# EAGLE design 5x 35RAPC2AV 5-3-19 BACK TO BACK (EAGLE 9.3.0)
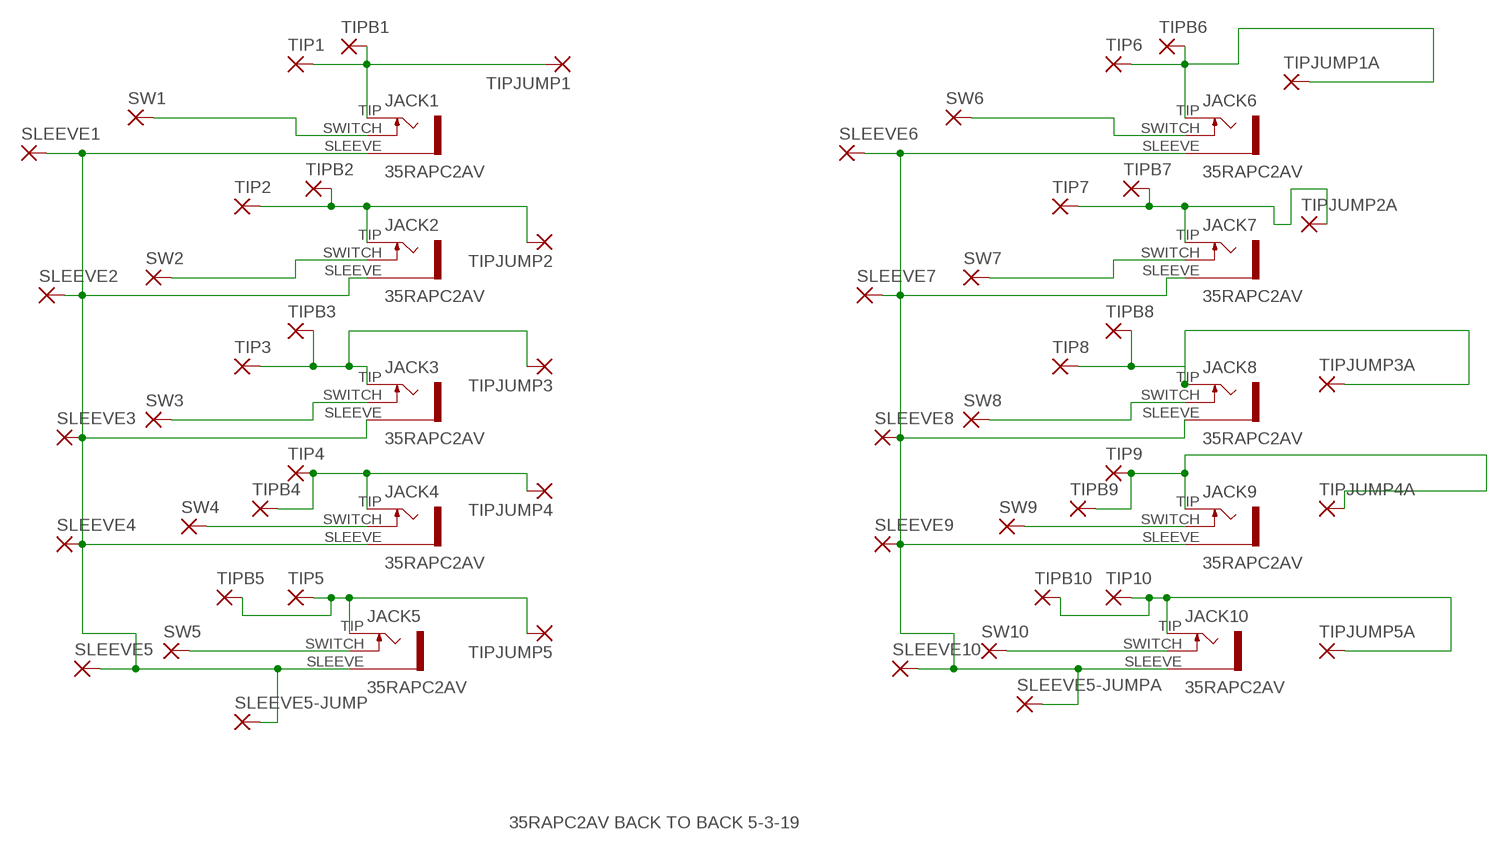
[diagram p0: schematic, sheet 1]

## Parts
JACK1  35RAPC2AV  [35RAPCVAV]
JACK2  35RAPC2AV  [35RAPCVAV]
JACK3  35RAPC2AV  [35RAPCVAV]
JACK4  35RAPC2AV  [35RAPCVAV]
JACK5  35RAPC2AV  [35RAPCVAV]
JACK6  35RAPC2AV  [35RAPCVAV]
JACK7  35RAPC2AV  [35RAPCVAV]
JACK8  35RAPC2AV  [35RAPCVAV]
JACK9  35RAPC2AV  [35RAPCVAV]
JACK10  35RAPC2AV  [35RAPCVAV]
SLEEVE1  2,54/1,1  [2,54/1,1]
SLEEVE2  2,54/1,1  [2,54/1,1]
SLEEVE3  2,54/1,1  [2,54/1,1]
SLEEVE4  2,54/1,1  [2,54/1,1]
SLEEVE5  2,54/1,1  [2,54/1,1]
SLEEVE5-JUMP  2,54/1,1  [2,54/1,1]
SLEEVE5-JUMPA  2,54/1,1  [2,54/1,1]
SLEEVE6  2,54/1,1  [2,54/1,1]
SLEEVE7  2,54/1,1  [2,54/1,1]
SLEEVE8  2,54/1,1  [2,54/1,1]
SLEEVE9  2,54/1,1  [2,54/1,1]
SLEEVE10  2,54/1,1  [2,54/1,1]
SW1  2,54/1,1  [2,54/1,1]
SW2  2,54/1,1  [2,54/1,1]
SW3  2,54/1,1  [2,54/1,1]
SW4  2,54/1,1  [2,54/1,1]
SW5  2,54/1,1  [2,54/1,1]
SW6  2,54/1,1  [2,54/1,1]
SW7  2,54/1,1  [2,54/1,1]
SW8  2,54/1,1  [2,54/1,1]
SW9  2,54/1,1  [2,54/1,1]
SW10  2,54/1,1  [2,54/1,1]
TIP1  2,54/1,1  [2,54/1,1]
TIP2  2,54/1,1  [2,54/1,1]
TIP3  2,54/1,1  [2,54/1,1]
TIP4  2,54/1,1  [2,54/1,1]
TIP5  2,54/1,1  [2,54/1,1]
TIP6  2,54/1,1  [2,54/1,1]
TIP7  2,54/1,1  [2,54/1,1]
TIP8  2,54/1,1  [2,54/1,1]
TIP9  2,54/1,1  [2,54/1,1]
TIP10  2,54/1,1  [2,54/1,1]
TIPB1  2,54/1,1  [2,54/1,1]
TIPB2  2,54/1,1  [2,54/1,1]
TIPB3  2,54/1,1  [2,54/1,1]
TIPB4  2,54/1,1  [2,54/1,1]
TIPB5  2,54/1,1  [2,54/1,1]
TIPB6  2,54/1,1  [2,54/1,1]
TIPB7  2,54/1,1  [2,54/1,1]
TIPB8  2,54/1,1  [2,54/1,1]
TIPB9  2,54/1,1  [2,54/1,1]
TIPB10  2,54/1,1  [2,54/1,1]
TIPJUMP1  2,54/1,1  [2,54/1,1]
TIPJUMP1A  2,54/1,1  [2,54/1,1]
TIPJUMP2  2,54/1,1  [2,54/1,1]
TIPJUMP2A  2,54/1,1  [2,54/1,1]
TIPJUMP3  2,54/1,1  [2,54/1,1]
TIPJUMP3A  2,54/1,1  [2,54/1,1]
TIPJUMP4  2,54/1,1  [2,54/1,1]
TIPJUMP4A  2,54/1,1  [2,54/1,1]
TIPJUMP5  2,54/1,1  [2,54/1,1]
TIPJUMP5A  2,54/1,1  [2,54/1,1]

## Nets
N$2: JACK1.SWITCH SW1.1(P)
N$3: JACK1.SLEEVE JACK2.SLEEVE JACK3.SLEEVE JACK4.SLEEVE JACK5.SLEEVE SLEEVE1.1(P) SLEEVE2.1(P) SLEEVE3.1(P) SLEEVE4.1(P) SLEEVE5-JUMP.1(P) SLEEVE5.1(P)
N$4: JACK2.TIP TIP2.1(P) TIPB2.1(P) TIPJUMP2.1(P)
N$5: JACK6.TIP TIP6.1(P) TIPB6.1(P) TIPJUMP1A.1(P)
N$6: JACK6.SWITCH SW6.1(P)
N$7: JACK6.SLEEVE JACK7.SLEEVE JACK8.SLEEVE JACK9.SLEEVE JACK10.SLEEVE SLEEVE5-JUMPA.1(P) SLEEVE6.1(P) SLEEVE7.1(P) SLEEVE8.1(P) SLEEVE9.1(P) SLEEVE10.1(P)
N$8: JACK3.SWITCH SW3.1(P)
N$9: JACK3.TIP TIP3.1(P) TIPB3.1(P) TIPJUMP3.1(P)
N$10: JACK4.TIP TIP4.1(P) TIPB4.1(P) TIPJUMP4.1(P)
N$11: JACK4.SWITCH SW4.1(P)
N$12: JACK7.TIP TIP7.1(P) TIPB7.1(P) TIPJUMP2A.1(P)
N$13: JACK5.TIP TIP5.1(P) TIPB5.1(P) TIPJUMP5.1(P)
N$14: JACK5.SWITCH SW5.1(P)
N$15: JACK8.SWITCH SW8.1(P)
N$16: JACK8.TIP TIP8.1(P) TIPB8.1(P) TIPJUMP3A.1(P)
N$17: JACK9.TIP TIP9.1(P) TIPB9.1(P) TIPJUMP4A.1(P)
N$18: JACK9.SWITCH SW9.1(P)
N$19: JACK10.TIP TIP10.1(P) TIPB10.1(P) TIPJUMP5A.1(P)
N$20: JACK10.SWITCH SW10.1(P)
SW1: JACK7.SWITCH SW7.1(P)
SW2: JACK2.SWITCH SW2.1(P)
TIP1: JACK1.TIP TIP1.1(P) TIPB1.1(P) TIPJUMP1.1(P)

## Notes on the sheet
- 35RAPC2AV BACK TO BACK 5-3-19

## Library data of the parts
JACK1-JACK10 = MusicThingModular-CL:35RAPC2AV: Switchcraft 35RAPC2AV jack
SLEEVE1-SLEEVE5 SLEEVE5-JUMP SLEEVE5-JUMPA SLEEVE6-SLEEVE10 SW1-SW10 TIP1-TIP10 TIPB1-TIPB10 TIPJUMP1 TIPJUMP1A TIPJUMP2 TIPJUMP2A TIPJUMP3 TIPJUMP3A TIPJUMP4 TIPJUMP4A TIPJUMP5 TIPJUMP5A = wirepad:2,54/1,1: THROUGH-HOLE PAD

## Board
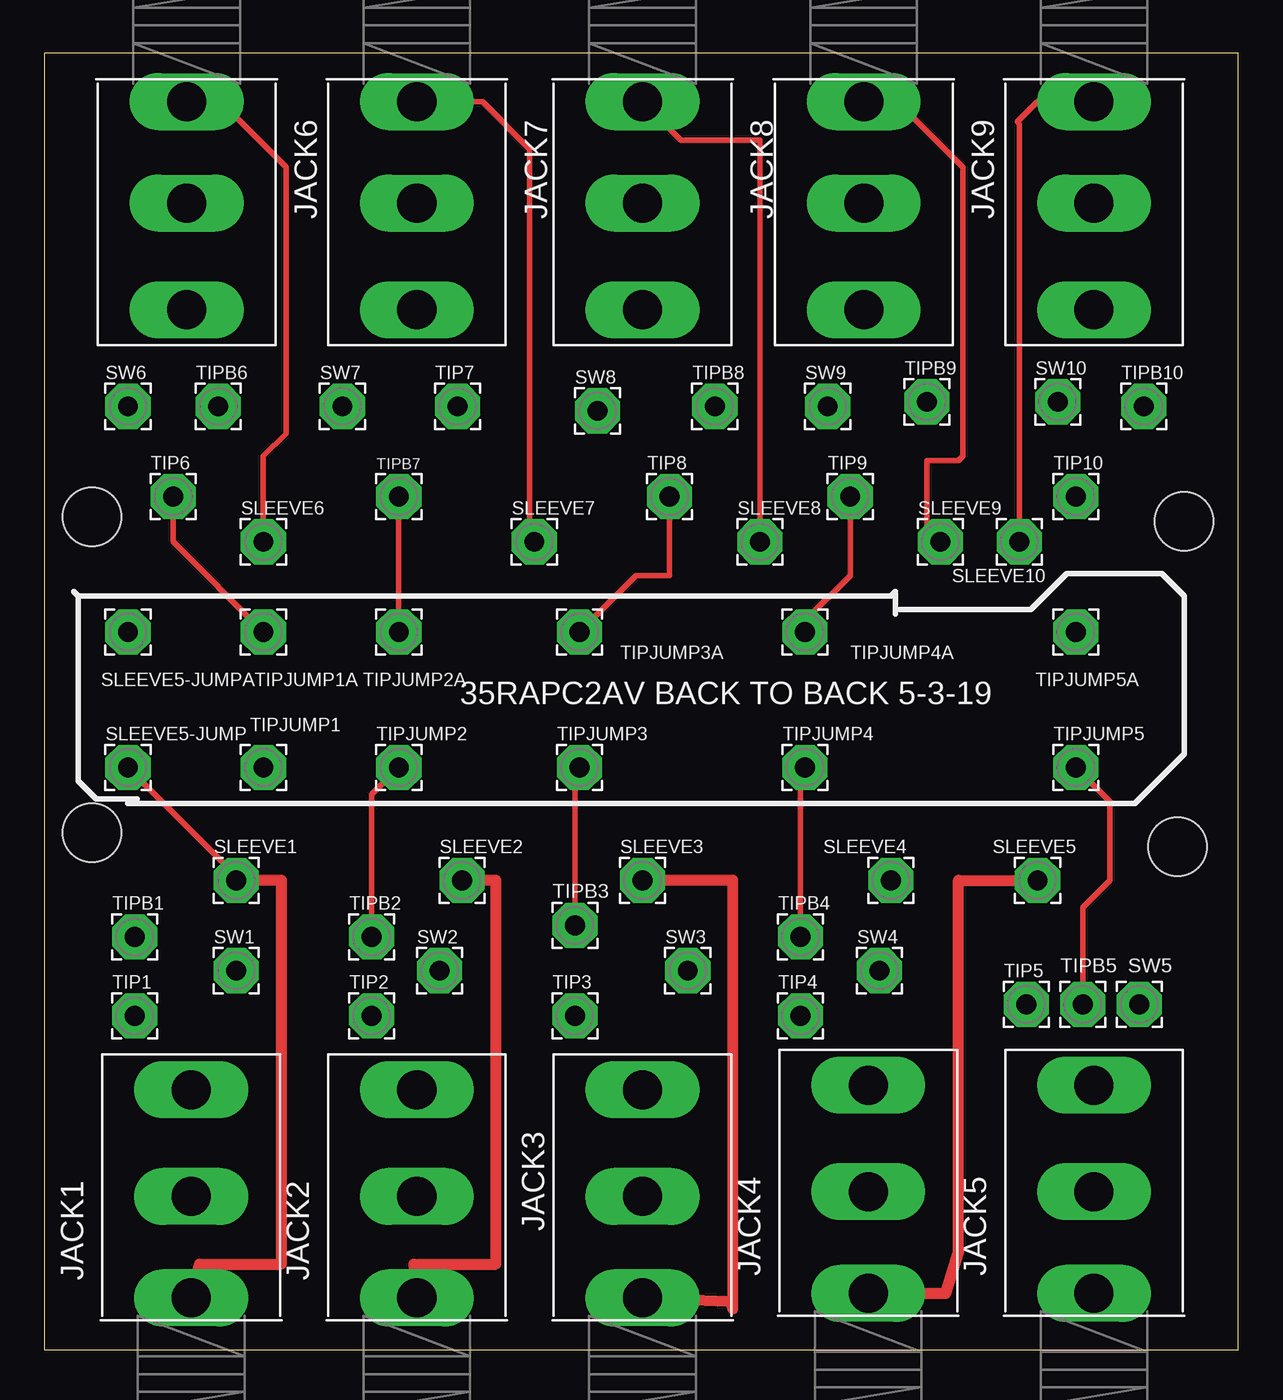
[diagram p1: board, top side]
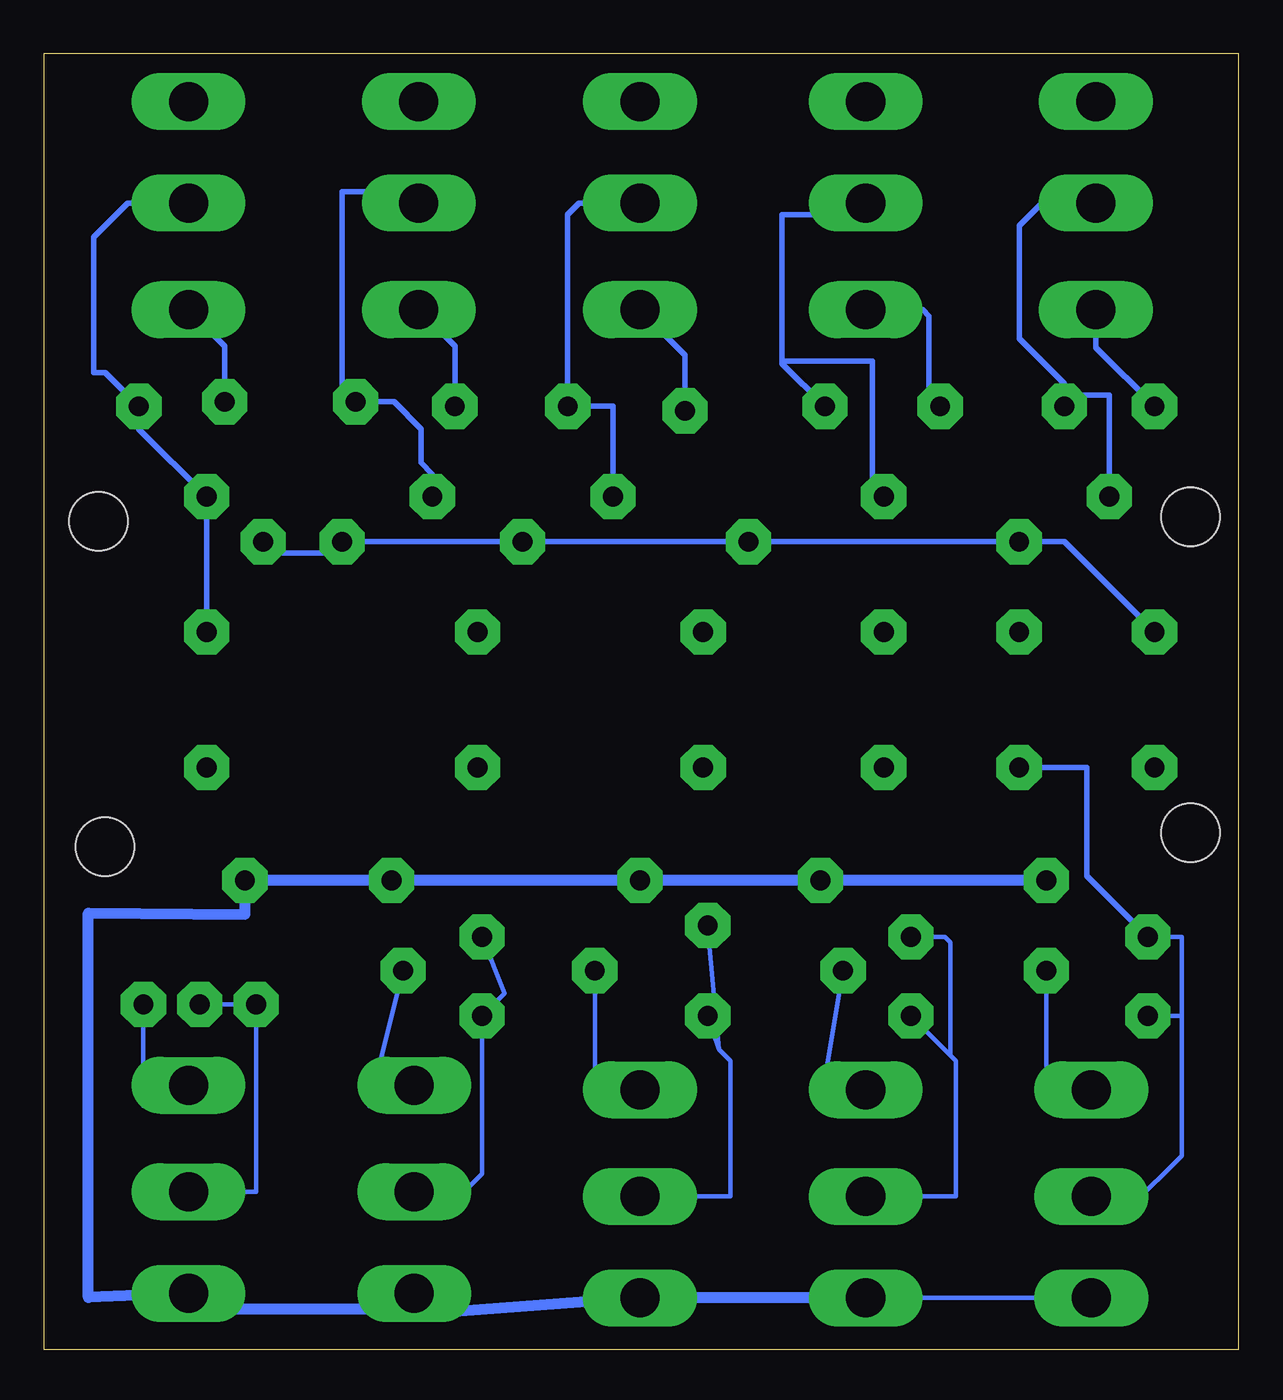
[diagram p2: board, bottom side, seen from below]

Size 67.16 x 72.95 mm. Coordinates in mm from the lower left corner, seen from the top.
Outline: 0,0 67.16,0 67.16,72.95 0,72.95 0,0
Copper layers (1*16): Top 0.035mm / dielectric 1.5mm / Bottom 0.035mm
Design rules "default": minimum track width 6mil, minimum drill 0.35mm, track to track 6mil, track to pad 6mil, pad to pad 6mil, via to via 6mil, smd to smd 6mil, copper to edge 40mil, drill to drill 6mil, minimum pad ring 10mil, minimum via ring 8mil, stop-mask expansion 4mil, vias tented up to drill 0mil, thermal gap 10mil
Holes 3.3 mm at 2.67,29.08 63.75,28.32 2.67,46.86 64.13,46.61

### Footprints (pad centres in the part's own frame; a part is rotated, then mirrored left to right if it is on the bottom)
35RAPCVAV = drill 2.2 pad 2.184 long: SLEEVE 0,-5.715; SWITCH 0,6; TIP 0,0
2,54/1,1 = drill 1.118 pad 2.54 octagon: 1 0,0

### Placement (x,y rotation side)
JACK1  8.25,8.64 0 top
JACK2  20.96,8.64 0 top
JACK3  33.66,8.64 0 top
JACK4  46.35,8.89 0 top
JACK5  59.05,8.89 0 top
JACK6  8,64.52 180 top
JACK7  20.96,64.52 180 top
JACK8  33.66,64.52 180 top
JACK9  46.1,64.52 180 top
JACK10  59.05,64.52 180 top
SLEEVE1  10.79,26.42 0 top
SLEEVE2  23.5,26.42 0 top
SLEEVE3  33.66,26.42 0 top
SLEEVE4  47.62,26.42 0 top
SLEEVE5  55.88,26.42 0 top
SLEEVE5-JUMP  4.7,32.77 0 top
SLEEVE5-JUMPA  4.7,40.39 0 top
SLEEVE6  12.32,45.47 0 top
SLEEVE7  27.56,45.47 0 top
SLEEVE8  40.26,45.47 0 top
SLEEVE9  50.42,45.47 0 top
SLEEVE10  54.86,45.47 0 top
SW1  10.79,21.34 0 top
SW2  22.22,21.34 0 top
SW3  36.19,21.34 0 top
SW4  46.99,21.34 0 top
SW5  61.59,19.43 0 top
SW6  4.7,53.09 0 top
SW7  16.76,53.09 0 top
SW8  31.11,52.83 0 top
SW9  44.07,53.09 0 top
SW10  57.02,53.34 0 top
TIP1  5.08,18.8 0 top
TIP2  18.42,18.8 0 top
TIP3  29.85,18.8 0 top
TIP4  42.55,18.8 0 top
TIP5  55.24,19.43 0 top
TIP6  7.24,48.01 0 top
TIP7  23.24,53.09 0 top
TIP8  35.18,48.01 0 top
TIP9  45.34,48.01 0 top
TIP10  58.04,48.01 0 top
TIPB1  5.08,23.24 0 top
TIPB2  18.42,23.24 0 top
TIPB3  29.85,23.88 0 top
TIPB4  42.55,23.24 0 top
TIPB5  58.42,19.43 0 top
TIPB6  9.78,53.09 0 top
TIPB7  19.94,48.01 0 top
TIPB8  37.72,53.09 0 top
TIPB9  49.66,53.34 0 top
TIPB10  61.85,53.09 0 top
TIPJUMP1  12.32,32.77 0 top
TIPJUMP1A  12.32,40.39 0 top
TIPJUMP2  19.94,32.77 0 top
TIPJUMP2A  19.94,40.39 0 top
TIPJUMP3  30.1,32.77 0 top
TIPJUMP3A  30.1,40.39 0 top
TIPJUMP4  42.8,32.77 0 top
TIPJUMP4A  42.8,40.39 0 top
TIPJUMP5  58.04,32.77 0 top
TIPJUMP5A  58.04,40.39 0 top

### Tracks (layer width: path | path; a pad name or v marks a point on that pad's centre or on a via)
N$2
  Bottom 0.254: SW1.1 10.79,13.72 9.55,13.72 JACK1.SWITCH
N$3
  Top 0.305: SLEEVE1.1 10.79,26.67 SLEEVE5-JUMP.1
  Top 0.61: JACK1.SLEEVE 8.73,4.83 13.33,4.83 13.33,26.42 SLEEVE1.1 | JACK2.SLEEVE 20.79,4.83 25.4,4.83 25.4,26.42 SLEEVE2.1 | JACK3.SLEEVE 38.55,2.73 38.73,2.29 38.73,26.42 SLEEVE3.1 | JACK4.SLEEVE 50.72,3.17 51.44,5.46 51.44,26.42 SLEEVE5.1
  Bottom 0.254: JACK1.SLEEVE JACK2.SLEEVE
  Bottom 0.61: SLEEVE1.1 SLEEVE2.1 SLEEVE3.1 SLEEVE4.1 SLEEVE5.1 55.88,24.51 64.7,24.58 64.7,2.96 JACK5.SLEEVE 58.3,2.29 46.35,2.29 44.89,2.1 JACK3.SLEEVE JACK2.SLEEVE
N$4
  Top 0.305: TIPB2.1 18.42,31.24 TIPJUMP2.1
  Bottom 0.254: TIP2.1 16.19,16.57 | 16.19,16.57 15.87,16.26 15.87,8.64 JACK2.TIP | 16.19,16.57 16.19,22.92 16.51,23.24 TIPB2.1
N$5
  Top 0.305: TIPJUMP1A.1 7.24,45.47 TIP6.1
  Bottom 0.305: TIP6.1 7.24,53.72 9.14,53.72 TIPB6.1 9.78,54.36 12.32,56.9 12.32,63.25 11.05,64.52 JACK6.TIP
N$6
  Bottom 0.305: SW6.1 8,56.39 JACK6.SWITCH
N$7
  Top 0.305: SLEEVE6.1 12.32,50.29 13.59,51.56 13.59,66.55 9.91,70.23 JACK6.SLEEVE | SLEEVE7.1 27.3,45.72 27.3,67.56 24.64,70.23 JACK7.SLEEVE | SLEEVE8.1 40.26,68.07 35.81,68.07 JACK8.SLEEVE | SLEEVE9.1 49.66,46.23 49.66,50.04 51.44,50.04 51.69,50.29 51.69,66.55 48.01,70.23 JACK9.SLEEVE | SLEEVE10.1 54.86,68.96 54.74,69.09 55.88,70.23 JACK10.SLEEVE
  Bottom 0.305: SLEEVE5-JUMPA.1 9.78,45.47 SLEEVE6.1 SLEEVE7.1 SLEEVE8.1 SLEEVE9.1 51.05,44.83 54.23,44.83 SLEEVE10.1
N$8
  Bottom 0.254: SW3.1 36.19,13.72 34.95,13.72 JACK3.SWITCH
N$9
  Top 0.305: TIPB3.1 29.85,32.51 TIPJUMP3.1
  Bottom 0.254: 29.21,16.89 TIP3.1 | JACK3.TIP 28.57,8.64 28.57,16.26 29.21,16.89 | 29.21,16.89 TIPB3.1
N$10
  Top 0.305: TIPB4.1 42.55,32.51 TIPJUMP4.1
  Bottom 0.254: JACK4.TIP 43.56,8.89 42.55,9.91 TIP4.1 41.27,20.07 TIPB4.1
N$11
  Bottom 0.254: SW4.1 48.89,13.72 48.01,13.72 JACK4.SWITCH
N$12
  Top 0.305: TIPJUMP2A.1 TIPB7.1
  Bottom 0.305: TIPB7.1 20.57,48.64 20.57,55.63 25.65,55.63 | 25.65,55.63 25.65,63.88 21.21,63.88 20.57,64.52 JACK7.TIP | TIP7.1 25.65,55.5 25.65,55.63
N$13
  Top 0.305: TIPB5.1 58.42,24.89 59.94,26.42 59.94,30.86 TIPJUMP5.1
  Bottom 0.254: JACK5.TIP 55.24,8.89 TIP5.1 TIPB5.1
N$14
  Bottom 0.254: SW5.1 61.59,13.72 60.71,13.72 JACK5.SWITCH
N$15
  Bottom 0.305: SW8.1 31.11,55.98 JACK8.SWITCH
N$16
  Top 0.305: TIPJUMP3A.1 33.27,43.56 35.18,43.56 TIP8.1
  Bottom 0.305: TIP8.1 35.18,53.09 TIPB8.1 37.72,63.88 37.08,64.52 JACK8.TIP
N$17
  Top 0.305: TIPJUMP4A.1 42.8,41.02 45.34,43.56 TIP9.1
  Bottom 0.305: TIP9.1 45.34,49.28 45.97,49.91 45.97,51.82 47.5,53.34 TIPB9.1 50.42,54.1 50.42,65.15 46.74,65.15 JACK9.TIP
N$18
  Bottom 0.305: SW9.1 44.07,56.48 JACK9.SWITCH
N$19
  Bottom 0.305: JACK10.TIP 62.48,64.52 64.39,62.61 64.39,54.99 63.75,54.99 TIPB10.1 61.85,51.82 TIP10.1 TIPJUMP5A.1
N$20
  Bottom 0.305: SW10.1 57.02,56.48 JACK10.SWITCH
SW1
  Bottom 0.305: SW7.1 17.4,53.72 17.4,58.17 17.75,58.52 JACK7.SWITCH
SW2
  Bottom 0.254: SW2.1 23.5,13.72 23.11,14.1 JACK2.SWITCH
TIP1
  Bottom 0.254: JACK1.TIP 6,8.1 3.18,10.92 3.18,18.8 | 3.18,18.8 TIP1.1 | 3.18,18.8 3.18,23.24 TIPB1.1
  Bottom 0.305: TIPB1.1 8.51,26.67 8.51,32.77 TIPJUMP1.1

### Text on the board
tNames: 35RAPC2AV BACK TO BACK 5-3-19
